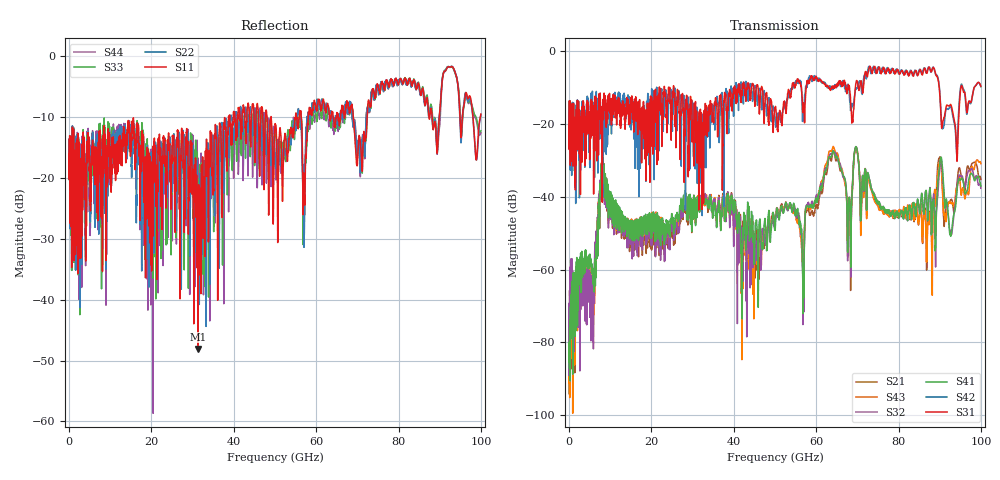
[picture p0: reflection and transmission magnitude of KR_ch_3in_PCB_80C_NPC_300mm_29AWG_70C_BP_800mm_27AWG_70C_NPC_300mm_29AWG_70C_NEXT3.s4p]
# GHz S RI R 45
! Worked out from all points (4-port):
!   4000 points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, 25 MHz to 100 GHz, reference 45 ohm
!   strongest paths, dB at 25 MHz, 25.02 GHz, 50.02 GHz, 75.03 GHz, 100 GHz:
!     S31: -20.0, -15.0, -15.7, -5.0, -9.6
!     S42: -20.0, -17.9, -18.0, -4.4, -9.7
!     S41: -87.0, -46.1, -49.1, -41.7, -37.0
!     S32: -89.0, -46.8, -46.9, -41.8, -37.6
!     S43: -89.5, -47.4, -46.0, -42.0, -30.9
!     S21: -94.1, -49.7, -47.2, -41.9, -35.2
!   lowest |S11| = -48.1 dB at 31.32 GHz (marker M1), VSWR 1.01, Z = 44.6 - j0.00134 ohm
!   |S11| at or under -10 dB: start of sweep to 38.73 GHz; 49.08 GHz to 54.98 GHz (5.895 GHz wide, 11.3 % of centre); 69.01 GHz to 72.38 GHz (3.365 GHz wide, 4.76 % of centre)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
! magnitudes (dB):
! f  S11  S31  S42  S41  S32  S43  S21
! 25 MHz  -16.0  -20.0  -20.0  -87.0  -89.0  -89.5  -94.1
! 5.9 GHz  -14.7  -20.1  -18.5  -63.8  -73.7  -78.4  -75.2
! 8.225 GHz  -14.7  -14.0  -22.2  -29.6  -29.8  -29.3  -30.1
! 31.32 GHz  -48.1  -21.3  -21.7  -42.6  -42.3  -41.8  -42.1
! 56.67 GHz  -16.7  -14.7  -19.3  -59.2  -58.3  -57.8  -57.2
! 63.92 GHz  -9.3  -9.6  -10.4  -27.8  -28.0  -26.9  -28.4
! 100 GHz  -9.5  -9.6  -9.7  -37.0  -37.6  -30.9  -35.2
